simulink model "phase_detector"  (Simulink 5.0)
settings: Solver=ode4  StartTime=0.0  StopTime=10  FixedStep=0.001  RelTol=1e-6

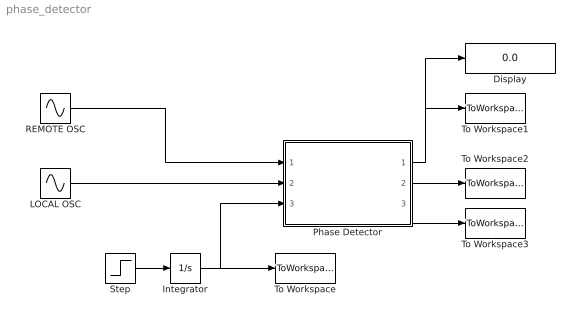
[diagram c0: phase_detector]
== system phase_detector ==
  Display : Display
  Integrator : Integrator
  LOCAL OSC : Sin  Frequency=2*pi*1  SampleTime=0
  Phase Detector : Subsystem
  REMOTE OSC : Sin  Frequency=2*pi*1.01  SampleTime=0
  Step : Step  Time=0  SampleTime=0
  To Workspace : ToWorkspace  VariableName=time  SampleTime=-1  SaveFormat=Array
  To Workspace1 : ToWorkspace  VariableName=output  SampleTime=-1  SaveFormat=Array
  To Workspace2 : ToWorkspace  VariableName=remote  SampleTime=-1  SaveFormat=Array
  To Workspace3 : ToWorkspace  VariableName=local  SampleTime=-1  SaveFormat=Array
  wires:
  Step/1 -> Integrator/1
  Integrator/1 -> To Workspace/1, Phase Detector/3(time)
  Phase Detector/1(output) -> Display/1, To Workspace1/1
  Phase Detector/2(remote) -> To Workspace2/1
  Phase Detector/3(local) -> To Workspace3/1
  REMOTE OSC/1 -> Phase Detector/1(REMOTE)
  LOCAL OSC/1 -> Phase Detector/2(LOCAL)

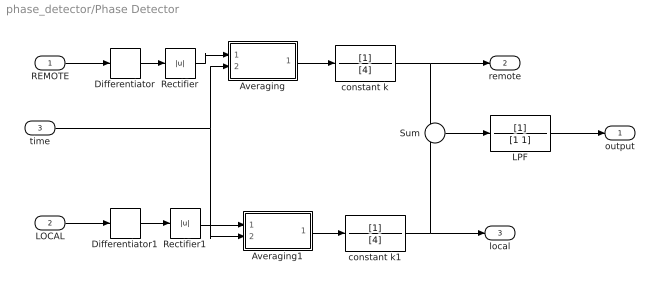
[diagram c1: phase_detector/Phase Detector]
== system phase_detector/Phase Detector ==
  REMOTE : Inport
  LOCAL : Inport  Port=2
  time : Inport  Port=3
  Averaging : Subsystem
  Averaging1 : Subsystem
  Differentiator : Derivative
  Differentiator1 : Derivative
  LPF : TransferFcn  Denominator=[1 1]
  Rectifier : Abs
  Rectifier1 : Abs
  Sum : Sum  Inputs=+-
  constant k : TransferFcn  Denominator=[4]
  constant k1 : TransferFcn  Denominator=[4]
  output : Outport
  remote : Outport  Port=2
  local : Outport  Port=3
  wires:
  time/1 -> Averaging/2(time), Averaging1/2(time)
  Differentiator/1 -> Rectifier/1
  Differentiator1/1 -> Rectifier1/1
  Sum/1 -> LPF/1
  Rectifier/1 -> Averaging/1(In1)
  Averaging/1(Out1) -> constant k/1
  Rectifier1/1 -> Averaging1/1(In1)
  Averaging1/1(Out1) -> constant k1/1
  LPF/1 -> output/1
  REMOTE/1 -> Differentiator/1
  LOCAL/1 -> Differentiator1/1
  constant k/1 -> remote/1, Sum/1
  constant k1/1 -> local/1, Sum/2

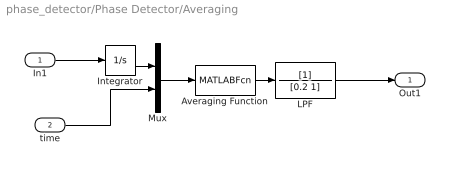
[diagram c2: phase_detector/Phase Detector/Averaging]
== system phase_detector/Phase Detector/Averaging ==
  In1 : Inport
  time : Inport  Port=2
  Averaging Function : MATLABFcn  MATLABFcn=rata2
  Integrator : Integrator
  LPF : TransferFcn  Denominator=[0.2 1]
  Mux : Mux  Inputs=2
  Out1 : Outport
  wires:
  In1/1 -> Integrator/1
  time/1 -> Mux/2
  Integrator/1 -> Mux/1
  Mux/1 -> Averaging Function/1
  Averaging Function/1 -> LPF/1
  LPF/1 -> Out1/1

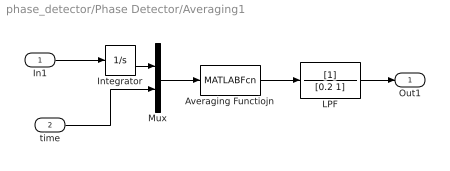
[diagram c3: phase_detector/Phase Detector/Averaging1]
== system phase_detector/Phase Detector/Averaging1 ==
  In1 : Inport
  time : Inport  Port=2
  Averaging Functiojn : MATLABFcn  MATLABFcn=rata2
  Integrator : Integrator
  LPF : TransferFcn  Denominator=[0.2 1]
  Mux : Mux  Inputs=2
  Out1 : Outport
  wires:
  In1/1 -> Integrator/1
  time/1 -> Mux/2
  Integrator/1 -> Mux/1
  Mux/1 -> Averaging Functiojn/1
  Averaging Functiojn/1 -> LPF/1
  LPF/1 -> Out1/1
